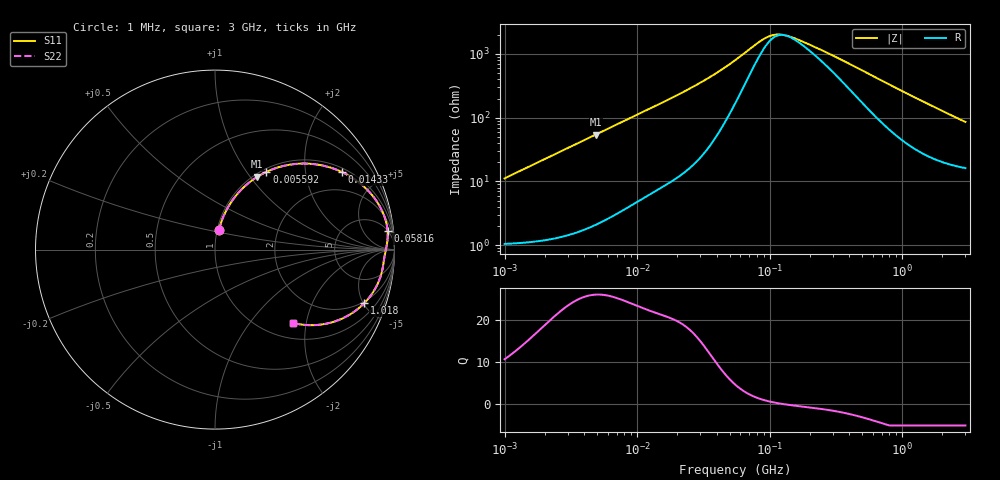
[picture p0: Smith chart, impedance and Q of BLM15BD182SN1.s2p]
! BLM15BD182SN1
# Hz S RI R 50
!Freq.(Hz) S11(Real) S11(Imag) S21(Real) S21(Imag) S12(Real) S12(Imag) S22(Real) S22(Imag)
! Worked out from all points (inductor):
!   401 points, 1 MHz to 3 GHz, reference 50 ohm
!   read as one part in series: L = 1.78 uH near 1.041 MHz
!   highest Q = 25.9 at 4.861 MHz (marker M1), where L = 1.77 uH
!   self-resonance near 129.8 MHz
!   S11 on the Smith chart (normalised r, x): 1 MHz: 1.02, +0.22; 5.592 MHz: 1.05, +1.24; 14.33 MHz: 1.15, +3.18; 58.16 MHz: 5, +17; 1.018 GHz: 1.86, -5.06; 3 GHz: 1.32, -1.68
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1000000  0.0223 0.108  0.9777 -0.108  0.9777 -0.108  0.0223 0.108
2182827  0.0663 0.2247  0.9337 -0.2247  0.9337 -0.2247  0.0663 0.2247
3823119  0.1635 0.3505  0.8365 -0.3505  0.8365 -0.3505  0.1635 0.3505
4861065  0.2354 0.4054  0.7646 -0.4054  0.7646 -0.4054  0.2354 0.4054
5592179  0.2868 0.4334  0.7132 -0.4334  0.7132 -0.4334  0.2868 0.4334
8861669  0.4923 0.4795  0.5077 -0.4795  0.5077 -0.4795  0.4923 0.4795
1.432659e7  0.7084 0.4318  0.2916 -0.4318  0.2916 -0.4318  0.7084 0.4318
1.461624e7  0.7163 0.428  0.2837 -0.428  0.2837 -0.428  0.7163 0.428
1.973457e7  0.819 0.3605  0.181 -0.3605  0.181 -0.3605  0.819 0.3605
2.718395e7  0.8949 0.2778  0.1051 -0.2778  0.1051 -0.2778  0.8949 0.2778
3.897472e7  0.9429 0.1877  0.0571 -0.1877  0.0571 -0.1877  0.9429 0.1877
5.477226e7  0.9606 0.1153  0.0394 -0.1153  0.0394 -0.1153  0.9606 0.1153
5.816196e7  0.9617 0.1042  0.0383 -0.1042  0.0383 -0.1042  0.9617 0.1042
8.679508e7  0.9599 0.0431  0.0401 -0.0431  0.0401 -0.0431  0.9599 0.0431
1.081723e8  0.9555 0.0179  0.0445 -0.0179  0.0445 -0.0179  0.9555 0.0179
1.375402e8  0.9505 -0.00527  0.0495 0.00527  0.0495 0.00527  0.9505 -0.00527
2.094008e8  0.9436 -0.0422  0.0564 0.0422  0.0564 0.0422  0.9436 -0.0422
4.219165e8  0.9299 -0.1233  0.0701 0.1233  0.0701 0.1233  0.9299 -0.1233
8.005644e8  0.8755 -0.245  0.1245 0.245  0.1245 0.245  0.8755 -0.245
1.017911e9  0.8305 -0.2996  0.1695 0.2996  0.1695 0.2996  0.8305 -0.2996
1.855641e9  0.6369 -0.4091  0.3631 0.4091  0.3631 0.4091  0.6369 -0.4091
3e9  0.4355 -0.4088  0.5645 0.4088  0.5645 0.4088  0.4355 -0.4088
